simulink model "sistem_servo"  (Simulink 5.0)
settings: Solver=ode4  StartTime=0.0  StopTime=10  FixedStep=0.01  RelTol=1e-3
libraries: simulink x1

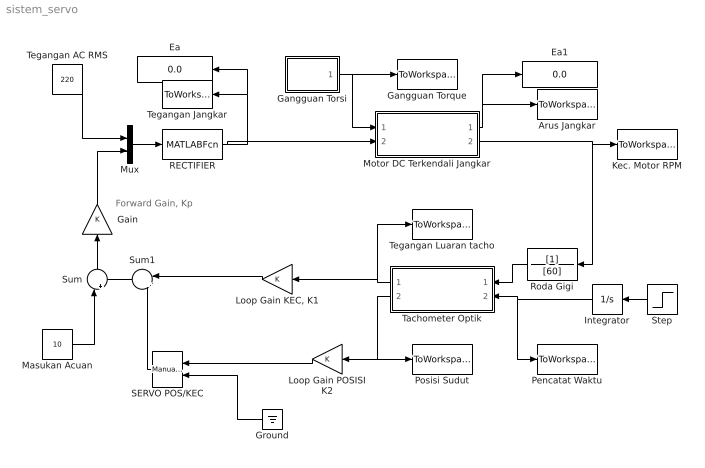
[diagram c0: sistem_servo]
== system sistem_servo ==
  note: Forward Gain, Kp
  Arus Jangkar : ToWorkspace  VariableName=arus  SampleTime=-1  SaveFormat=Array
  Ea : Display
  Ea1 : Display
  Gain : Gain  Orientation=up
  Gangguan Torque : ToWorkspace  VariableName=gangguan  SampleTime=-1  SaveFormat=Array
  Gangguan Torsi : Subsystem
  Ground : Ground  Orientation=left
  Integrator : Integrator  Orientation=left
  Kec. Motor RPM : ToWorkspace  VariableName=rpm  SampleTime=-1  SaveFormat=Array
  "Loop Gain KEC, K1" : Gain  Orientation=left
  Loop Gain POSISI K2 : Gain  Orientation=left
  Masukan Acuan : Constant  Value=10
  Motor DC Terkendali Jangkar : Subsystem
  Mux : Mux  Inputs=2
  Pencatat Waktu : ToWorkspace  VariableName=time  SampleTime=-1  SaveFormat=Array
  Posisi Sudut : ToWorkspace  VariableName=teta  SampleTime=-1  SaveFormat=Array
  RECTIFIER : MATLABFcn  MATLABFcn=rectifier
  Roda Gigi : TransferFcn  Orientation=left  Denominator=[60]
  SERVO POS/KEC : simulink/Signal Routing/Manual Switch  Orientation=left  sw=1  action=0
  Step : Step  Orientation=left  Time=0  SampleTime=0
  Sum : Sum  Orientation=up  Inputs=|+-
  Sum1 : Sum  Orientation=left  Inputs=|++
  Tachometer Optik : Subsystem  Orientation=left
  Tegangan AC RMS : Constant  Value=220
  Tegangan Jangkar : ToWorkspace  VariableName=tegangan  SampleTime=-1  SaveFormat=Array
  Tegangan Luaran tacho : ToWorkspace  VariableName=vout  SampleTime=-1  SaveFormat=Array
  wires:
  Sum/1 -> Gain/1
  Masukan Acuan/1 -> Sum/1
  Motor DC Terkendali Jangkar/1(ia(t)) -> Arus Jangkar/1, Ea1/1
  Motor DC Terkendali Jangkar/2(RPM) -> Kec. Motor RPM/1, Roda Gigi/1
  Roda Gigi/1 -> Tachometer Optik/1(In1)
  Tachometer Optik/1(Vo) -> Tegangan Luaran tacho/1, "Loop Gain KEC, K1"/1
  Tachometer Optik/2(Teta) -> Posisi Sudut/1, Loop Gain POSISI K2/1
  Sum1/1 -> Sum/2
  "Loop Gain KEC, K1"/1 -> Sum1/1
  SERVO POS/KEC/1 -> Sum1/2
  Loop Gain POSISI K2/1 -> SERVO POS/KEC/1
  Ground/1 -> SERVO POS/KEC/2
  Step/1 -> Integrator/1
  Integrator/1 -> Pencatat Waktu/1, Tachometer Optik/2(time)
  Gangguan Torsi/1(Out1) -> Motor DC Terkendali Jangkar/1(u(t)), Gangguan Torque/1
  Mux/1 -> RECTIFIER/1
  Tegangan AC RMS/1 -> Mux/1
  Gain/1 -> Mux/2
  RECTIFIER/1 -> Motor DC Terkendali Jangkar/2(ea(t)), Tegangan Jangkar/1, Ea/1

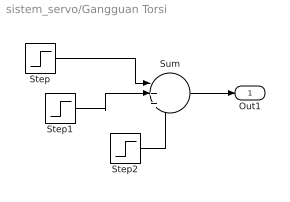
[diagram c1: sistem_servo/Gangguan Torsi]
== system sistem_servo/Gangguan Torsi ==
  Step : Step  Time=2  SampleTime=0
  Step1 : Step  Time=2.5  After=-2  SampleTime=0
  Step2 : Step  Time=2.75  SampleTime=0
  Sum : Sum  Inputs=|+++
  Out1 : Outport
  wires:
  Sum/1 -> Out1/1
  Step/1 -> Sum/1
  Step1/1 -> Sum/2
  Step2/1 -> Sum/3

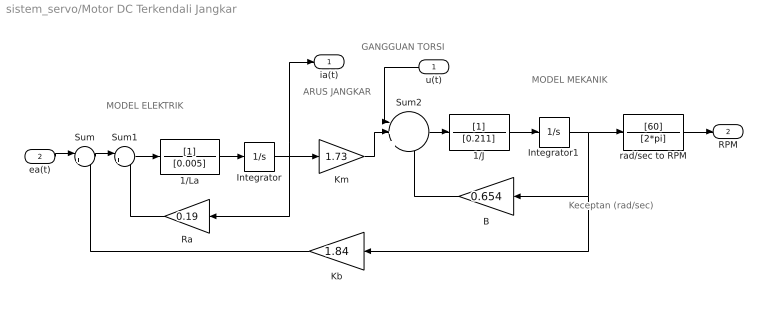
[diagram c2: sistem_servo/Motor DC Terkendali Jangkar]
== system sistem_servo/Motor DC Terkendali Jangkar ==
  note: Keceptan (rad/sec)
  note: MODEL ELEKTRIK
  note: MODEL MEKANIK
  note: GANGGUAN TORSI
  note: ARUS JANGKAR
  u(t) : Inport  Orientation=left
  ea(t) : Inport  Port=2
  1/J : TransferFcn  Denominator=[0.211]
  1/La : TransferFcn  Denominator=[0.005]
  B : Gain  Orientation=left  Gain=0.654
  Integrator : Integrator
  Integrator1 : Integrator
  Kb : Gain  Orientation=left  Gain=1.84
  Km : Gain  Gain=1.73
  Ra : Gain  Orientation=left  Gain=0.19
  Sum : Sum  Inputs=|+-
  Sum1 : Sum  Inputs=|+-
  Sum2 : Sum  Inputs=|++-
  rad/sec to RPM : TransferFcn  Numerator=[60]  Denominator=[2*pi]
  ia(t) : Outport
  RPM : Outport  Port=2
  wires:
  Sum/1 -> Sum1/1
  Sum1/1 -> 1/La/1
  1/La/1 -> Integrator/1
  Integrator/1 -> Km/1, Ra/1, ia(t)/1
  Kb/1 -> Sum/2
  ea(t)/1 -> Sum/1
  Ra/1 -> Sum1/2
  Integrator1/1 -> rad/sec to RPM/1, B/1, Kb/1
  rad/sec to RPM/1 -> RPM/1
  1/J/1 -> Integrator1/1
  Sum2/1 -> 1/J/1
  B/1 -> Sum2/3
  Km/1 -> Sum2/2
  u(t)/1 -> Sum2/1

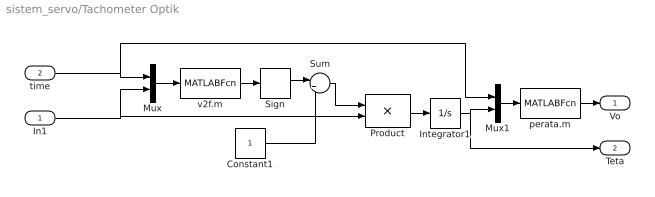
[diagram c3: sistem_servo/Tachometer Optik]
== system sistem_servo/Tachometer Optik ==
  In1 : Inport
  time : Inport  Port=2
  Constant1 : Constant
  Integrator1 : Integrator
  Mux : Mux  Inputs=2
  Mux1 : Mux  Inputs=2
  Product : Product
  Sign : Signum
  Sum : Sum  Inputs=|++
  perata.m : MATLABFcn  MATLABFcn=perata
  v2f.m : MATLABFcn  MATLABFcn=v2f
  Vo : Outport
  Teta : Outport  Port=2
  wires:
  time/1 -> Mux/1, Mux1/1
  Mux/1 -> v2f.m/1
  v2f.m/1 -> Sign/1
  Product/1 -> Integrator1/1
  Integrator1/1 -> Mux1/2, Teta/1
  Mux1/1 -> perata.m/1
  perata.m/1 -> Vo/1
  Sign/1 -> Sum/1
  Sum/1 -> Product/1
  Constant1/1 -> Sum/2
  In1/1 -> Product/2, Mux/2
